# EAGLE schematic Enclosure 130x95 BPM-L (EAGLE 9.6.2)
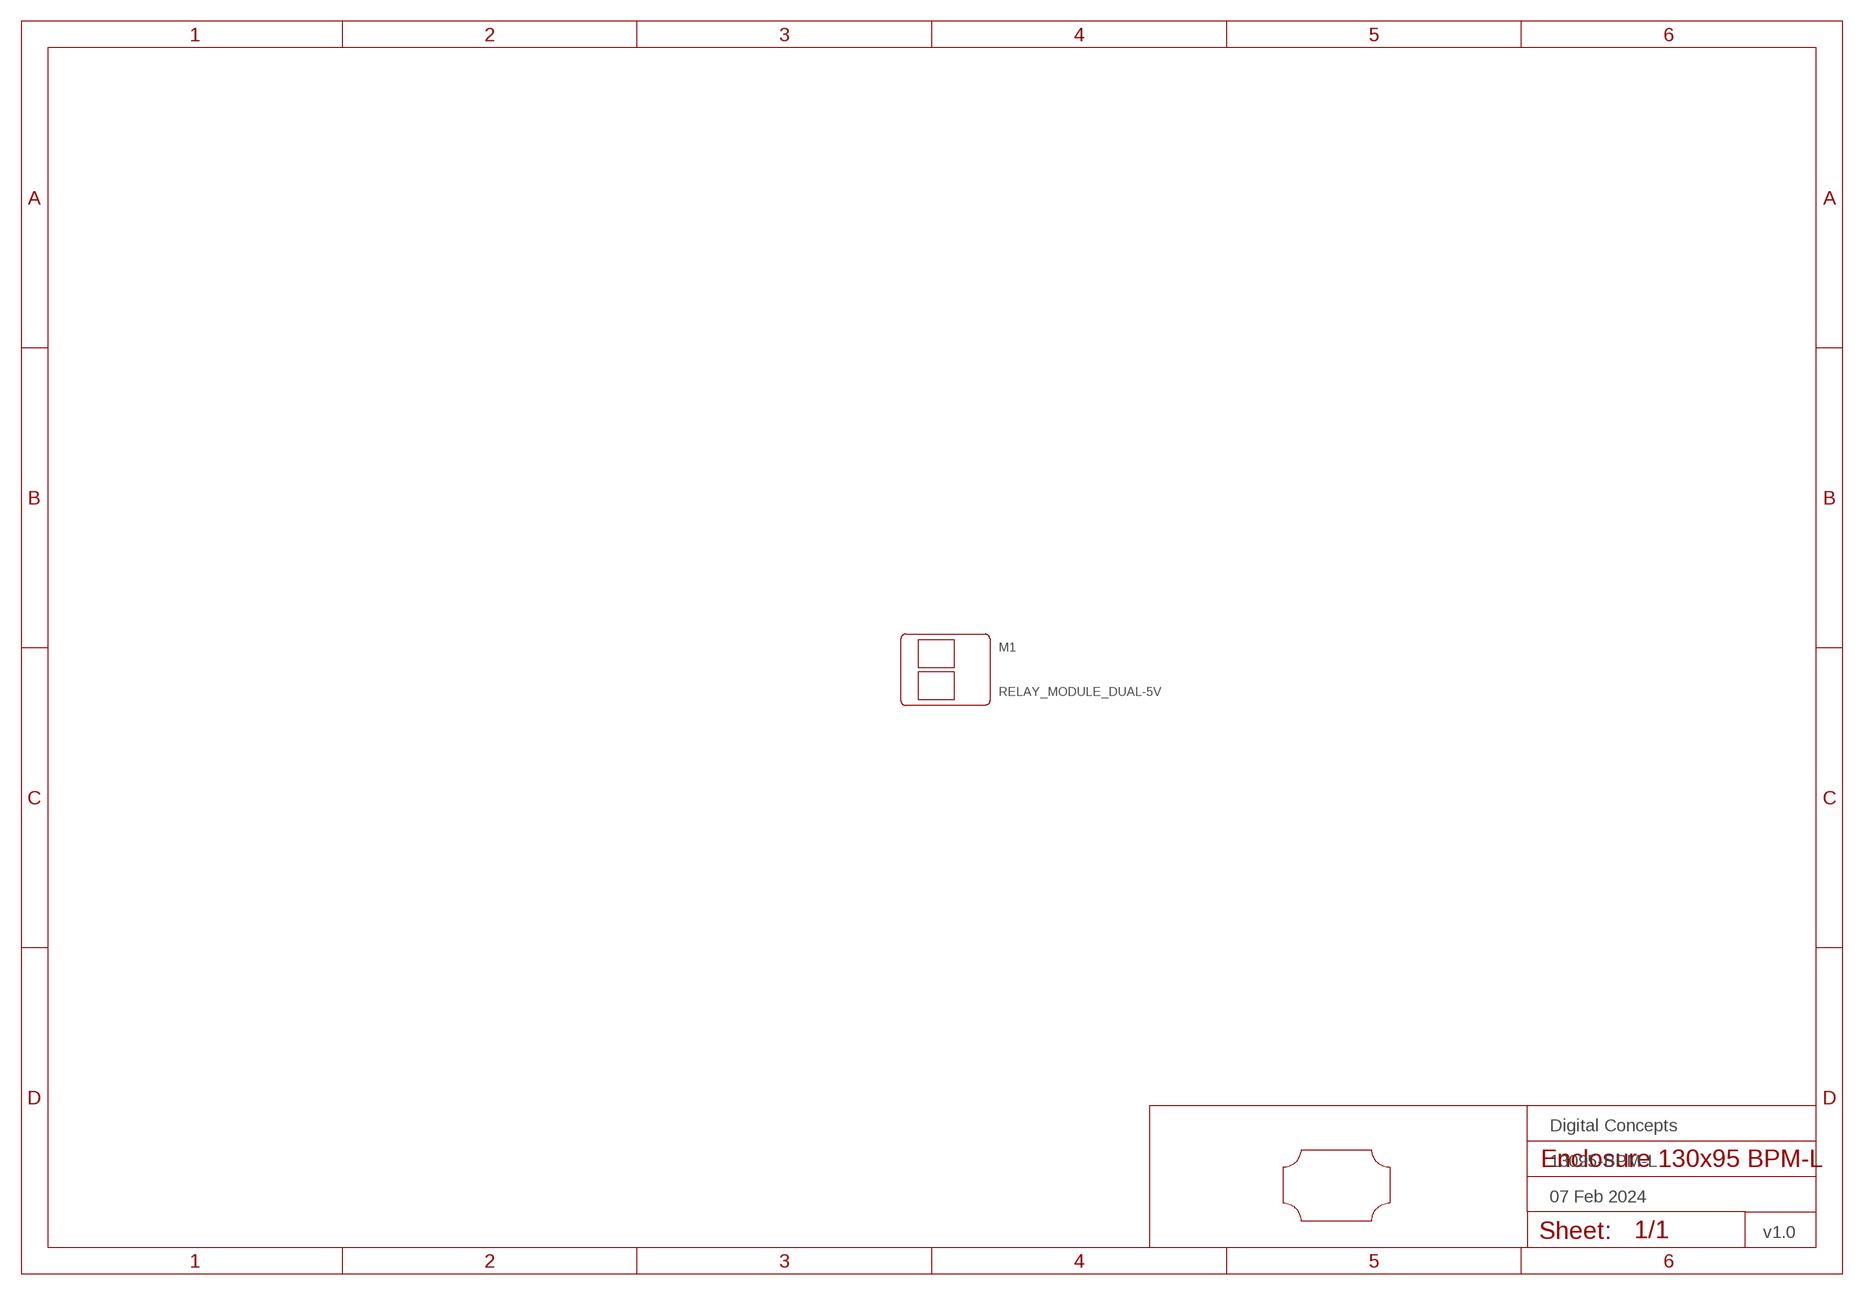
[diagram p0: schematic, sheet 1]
FRAME1 (FRAME-A4L-LOC): DATE: 07 Feb 2024; OWNER: Digital Concepts; TITLE: 13095-BPM-L; VERSION: v1.0

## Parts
M1  RELAY_MODULE_DUAL-5V  [RELAY-MODULE-DUAL-5V]
U$1  PCB-OUTLINE-130X95-MAX-LCM-H3  [PROTO-130X95-OUTLINE-MAX-LCM-H3]

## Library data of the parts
M1 = digitalconcepts:RELAY_MODULE_DUAL-5V: Dual Relay Module (5V)
U$1 = digitalconcepts:PCB-OUTLINE-130X95-MAX-LCM-H3: PCB Eagle Max-Left-Cropped outline for 130 x 95 enclosure (Horizontal format)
